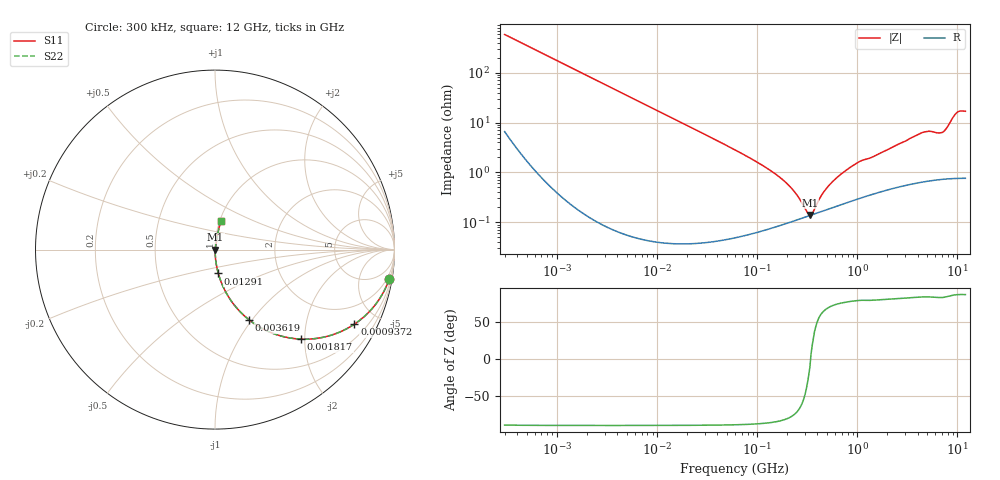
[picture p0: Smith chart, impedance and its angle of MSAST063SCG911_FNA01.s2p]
! MSAST063SCG911_FNA01  S-PARAMETER MODEL  ( General Type )
! Model Generated by TAIYO YUDEN Corporation (http://www.ty-top.com)
! Version 1.0
! TAIYO YUDEN Control No. 160830
! Copyright(c) 2016 TAIYO YUDEN CO.,LTD. All Rights Reserved.
! Product Description (link to TY-COMPAS)
! https://ds.yuden.co.jp/TYCOMPAS/or/detail?pn=MSAST063SCG911JFNA01&u=M
! Products Name : Multilayer Ceramic Capacitors
! Characteristics :
!  Capacitance : 910 pF , Rated Voltage : 25V , TCC : CG / C0G
!  Case Size : 0.6 x 0.3 / 0.024 x 0.012 [mm/inch] , Thickness : 0.3 / 0.012 [mm/inch]
!  (Conditions: Temperature = 25 degC , DC Bias Current/Voltage = 0A / 0V)
! External Node Assignments :
!  1  o---| |---o  2
! GND o---------o GND
! Frequency Range : 0.3MHz  -  12000MHz  [ 401 STEP ]
# MHz S RI R 50
! Freq[MHz].  S11 Real  S11 Imag  S21 Real  S21 Imag  S12 Real  S12 Imag  S22 Real  S22 Imag
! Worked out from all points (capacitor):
!   401 points, 300 kHz to 12 GHz, reference 50 ohm
!   read as one part in series: C = 910 pF near 316.3 kHz
!   lowest |Z| = 139 mohm at 335.7 MHz (marker M1)
!   series resonance near 341.3 MHz, so ESL is about 240 pH
!   S11 on the Smith chart (normalised r, x): 300 kHz: 1, -12; 937.2 kHz: 1.01, -3.73; 1.817 MHz: 1.00, -1.92; 3.619 MHz: 1.00, -0.97; 12.91 MHz: 1.00, -0.27; 12 GHz: 1.02, +0.34
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0.3  0.9697 -0.166  0.0303 0.166  0.0303 0.166  0.9697 -0.166
0.566559  0.9041 -0.2925  0.0959 0.2925  0.0959 0.2925  0.9041 -0.2925
0.937222  0.7764 -0.4155  0.2236 0.4155  0.2236 0.4155  0.7764 -0.4155
1.769972  0.494 -0.4992  0.506 0.4992  0.506 0.4992  0.494 -0.4992
1.817488  0.4808 -0.4988  0.5192 0.4988  0.5192 0.4988  0.4808 -0.4988
3.61914  0.1896 -0.3913  0.8104 0.3913  0.8104 0.3913  0.1896 -0.3913
10.44266  0.0276 -0.1626  0.9724 0.1626  0.9724 0.1626  0.0276 -0.1626
12.90781  0.0183 -0.1328  0.9817 0.1328  0.9817 0.1328  0.0183 -0.1328
60  0.00128 -0.0282  0.9987 0.0282  0.9987 0.0282  0.00128 -0.0282
119.4772  0.000859 -0.0129  0.9991 0.0129  0.9991 0.0129  0.000859 -0.0129
182.544  0.000951 -0.00688  0.999 0.00688  0.999 0.00688  0.000951 -0.00688
237.9135  0.00109 -0.00384  0.9989 0.00384  0.9989 0.00384  0.00109 -0.00384
335.7268  0.00137 -0.000268  0.9986 0.000268  0.9986 0.000268  0.00137 -0.000268
353.9943  0.00142 0.000468  0.9986 -0.000468  0.9986 -0.000468  0.00142 0.000468
461.3684  0.00172 0.00365  0.9983 -0.00365  0.9983 -0.00365  0.00172 0.00365
651.0506  0.00224 0.00814  0.9978 -0.00814  0.9978 -0.00814  0.00224 0.00814
1021.415  0.00319 0.0156  0.9968 -0.0156  0.9968 -0.0156  0.00319 0.0156
2088.533  0.00539 0.0292  0.9946 -0.0292  0.9946 -0.0292  0.00539 0.0292
4502.883  0.0103 0.0621  0.9897 -0.0621  0.9897 -0.0621  0.0103 0.0621
7064.448  0.0111 0.0619  0.9889 -0.0619  0.9889 -0.0619  0.0111 0.0619
9708.23  0.0299 0.1475  0.9701 -0.1475  0.9701 -0.1475  0.0299 0.1475
12000  0.0344 0.1611  0.9656 -0.1611  0.9656 -0.1611  0.0344 0.1611
